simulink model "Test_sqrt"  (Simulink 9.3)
settings: Solver=VariableStepAuto  StartTime=0.0  StopTime=4  RelTol=1e-3
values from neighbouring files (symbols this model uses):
  Tstep = 0.000050    (= 5e-05)    [TestOrthOsc_init.m]    (also in Test_PIDctrl_init.m = 0.0001)
libraries: libVishia_Ctrl x1

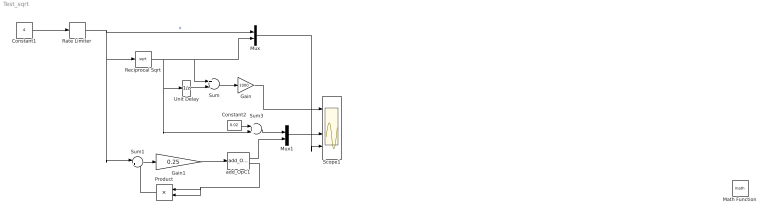
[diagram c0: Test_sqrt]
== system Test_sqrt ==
  Constant1 : Constant  Value=4  SampleTime=Tstep
  Constant2 : Constant  Value=0.02  SampleTime=Tstep
  Gain : Gain  Gain=1000
  Gain1 : Gain  Gain=0.25
  Math Function : Math
  Mux : Mux  Inputs=2
  Mux1 : Mux  Inputs=2
  Product : Product
  Rate Limiter : RateLimiter  SampleTimeMode=inherited
  Reciprocal Sqrt : Sqrt
  Scope1 : Scope  NumInputPorts=4
  Sum : Sum  Inputs=+-
  Sum1 : Sum  Inputs=|+-
  Sum3 : Sum
  Unit Delay : UnitDelay  SampleTime=-1  HasFrameUpgradeWarning=on
  add_OpC1 : libVishia_Ctrl/add_OpC  y0=0
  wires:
  Constant1/1 -> Rate Limiter/1
  Rate Limiter/1 -> Mux/1, Reciprocal Sqrt/1, Sum1/1  "x"
  Reciprocal Sqrt/1 -> Sum3/2, Unit Delay/1, Sum/1, Mux/2
  Mux/1 -> Scope1/4
  Unit Delay/1 -> Sum/2
  Sum/1 -> Gain/1
  Gain/1 -> Scope1/1
  Product/1 -> Sum1/2
  add_OpC1/2 -> Product/2, Product/1
  Sum1/1 -> Gain1/1
  add_OpC1/1 -> Mux1/2
  Gain1/1 -> add_OpC1/1
  Mux1/1 -> Scope1/3
  Constant2/1 -> Sum3/1
  Sum3/1 -> Mux1/1
